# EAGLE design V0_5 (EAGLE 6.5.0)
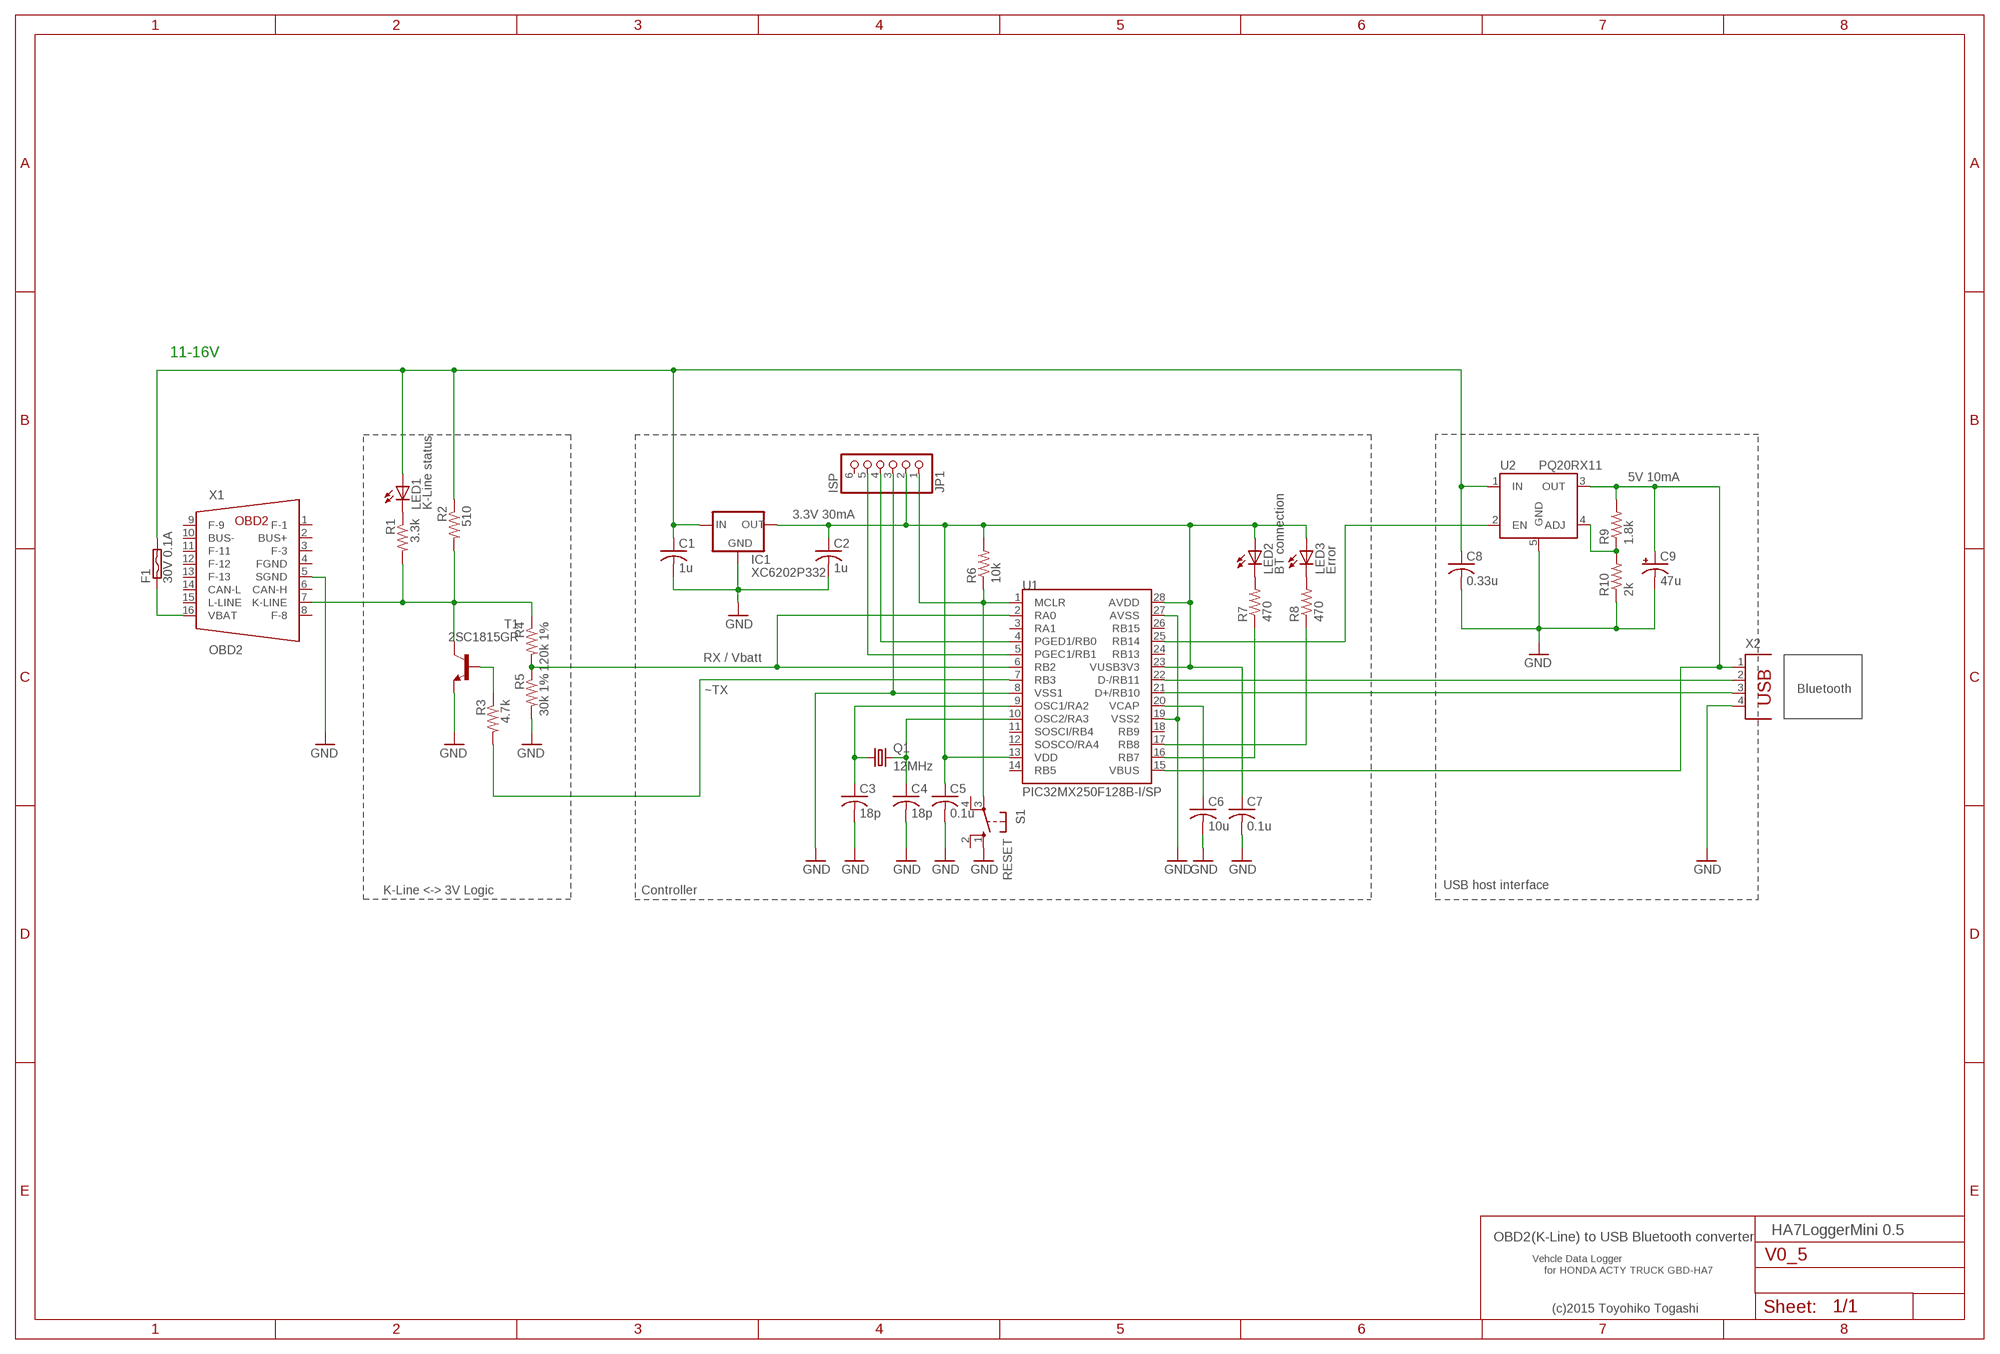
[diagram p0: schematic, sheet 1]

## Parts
C1  1u  C-US025-024X044  [C025-024X044]
C2  1u  C-US025-024X044  [C025-024X044]
C3  18p  C-US025-024X044  [C025-024X044]
C4  18p  C-US025-024X044  [C025-024X044]
C5  0.1u  C-US025-024X044  [C025-024X044]
C6  10u  C-US025-024X044  [C025-024X044]
C7  0.1u  C-US025-024X044  [C025-024X044]
C8  0.33u  C-US025-024X044  [C025-024X044]
C9  47u  CPOL-USE2.5-7  [E2,5-7]
F1  30V 0.1A  SMDH120  [SMD050F]
IC1  XC6202P332  78LXX  [78LXX]
JP1  ISP  PINHD-1X6  [1X06]
LED1  K-Line status  LED3MM  [LED3MM]
LED2  BT connection  LED3MM  [LED3MM]
LED3  Error  LED3MM  [LED3MM]
Q1  12MHz  CRYSTALHC49S  [HC49/S]
R1  3.3k  R-US_0204/5  [0204/5]
R2  510  R-US_0204/7  [0204/7]
R3  4.7k  R-US_0204/5  [0204/5]
R4  120k 1%  R-US_0204/7  [0204/7]
R5  30k 1%  R-US_0204/7  [0204/7]
R6  10k  R-US_0204/5  [0204/5]
R7  470  R-US_0204/5  [0204/5]
R8  470  R-US_0204/5  [0204/5]
R9  1.8k  R-US_0204/5  [0204/5]
R10  2k  R-US_0204/5  [0204/5]
S1  RESET  10-XX  [B3F-10XX]
T1  2SC1815GR  -NPN-TO92-ECB  [TO92-ECB]
U1  PIC32MX250F128B-I/SP  [DIL28-3]
U2  PQ20RX11  [L200S]
X1  OBD2  [2X08]
X2  PN87520  [PN87520]

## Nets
+5V: C9.+ R9.2 U1.15(VBUS) U2.3(OUT) X2.1
GND: C1.2 C2.2 C3.2 C4.2 C5.2 C6.2 C7.2 C8.2 C9.- IC1.GND JP1.3 R5.2 R10.1 S1.1(S) T1.E U1.8(VSS1) U1.19(VSS2) U1.27(AVSS) U2.5(GND) X1.5(SGND) X2.4
N$1: C3.1 Q1.1 U1.9(OSC1/RA2)
N$2: C4.1 Q1.2 U1.10(OSC2/RA3)
N$3: R7.1 U1.16(RB7)
N$4: JP1.4 U1.4(PGED1/RB0)
N$5: R3.2 U1.7(RB3)
N$6: R3.1 T1.B
N$7: JP1.5 U1.5(PGEC1/RB1)
N$8: C6.1 U1.20(VCAP)
N$9: U1.22(D-/RB11) X2.2
N$10: U1.21(D+/RB10) X2.3
N$11: LED2.K(C) R7.2
N$12: JP1.1 R6.1 S1.3(P) U1.1(MCLR)
N$15: LED3.K(C) R8.2
N$17: R8.1 U1.17(RB8)
N$18: F1.1 X1.16(VBAT)
N$20: R1.2 R2.2 R4.1 T1.C X1.7(K-LINE)
N$21: R4.2 R5.1 U1.2(RA0) U1.6(RB2)
N$22: LED1.K(C) R1.1
N$23: R9.1 R10.2 U2.4(ADJ)
N$24: U1.25(RB14) U2.2(EN)
N$26: C1.1 C8.1 F1.2 IC1.IN LED1.A R2.1 U2.1(IN)
N$32: C2.1 C5.1 C7.1 IC1.OUT JP1.2 LED2.A LED3.A R6.2 U1.13(VDD) U1.23(VUSB3V3) U1.28(AVDD)
Unconnected: JP1.6 S1.2(S1) S1.4(P1) U1.3(RA1) U1.11(SOSCI/RB4) U1.12(SOSCO/RA4) U1.14(RB5) U1.18(RB9) U1.24(RB13) U1.26(RB15) X1.1(F-1) X1.2(BUS+) X1.3(F-3) X1.6(CAN-H) X1.8(F-8) X1.9(F-9) X1.10(BUS-) X1.11(F-11) X1.12(F-12) X1.13(F-13) X1.14(CAN-L) X1.15(L-LINE)

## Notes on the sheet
- 11-16V
- 5V 10mA
- 3.3V 30mA
- RX / Vbatt
- ~TX | Bluetooth
- USB host interface
- K-Line <-> 3V Logic | Controller
- HA7LoggerMini 0.5
- OBD2(K-Line) to USB Bluetooth converter
- Vehcle Data Logger
- for HONDA ACTY TRUCK GBD-HA7
- (c)2015 Toyohiko Togashi

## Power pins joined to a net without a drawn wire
FGND: X1.4(FGND)

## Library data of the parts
C1-C8 = rcl:C-US: CAPACITOR, American symbol
C9 = rcl:CPOL-US: POLARIZED CAPACITOR, American symbol
F1 = switch-raychem:SMDH120: PolySwitch (TM) Resettable Device
IC1 = v-reg:78LXX: VOLTAGE REGULATOR
JP1 = pinhead:PINHD-1X6: PIN HEADER
LED1-LED3 = led:LED: LED
Q1 = crystal:CRYSTAL: CRYSTAL; OC_FARNELL: 1667008; OC_NEWARK: unknown
R1-R10 = rcl:R-US_: RESISTOR, American symbol
S1 = switch-omron:10-XX: OMRON SWITCH; MPN: B3F-1000; OC_FARNELL: 176432; OC_NEWARK: 36M3542
T1 = transistor:*-NPN-: NPN Transistror BF959 corrected 2008.03.06
U1 = TOG.rpt:PIC32MX250F128B
U2 = TOG:PQ20RX
X1 = TOG:OBD2: OBD2 Connecter
X2 = con-berg:PN87520: BERG USB connector; OC_FARNELL: unknown; OC_NEWARK: unknown

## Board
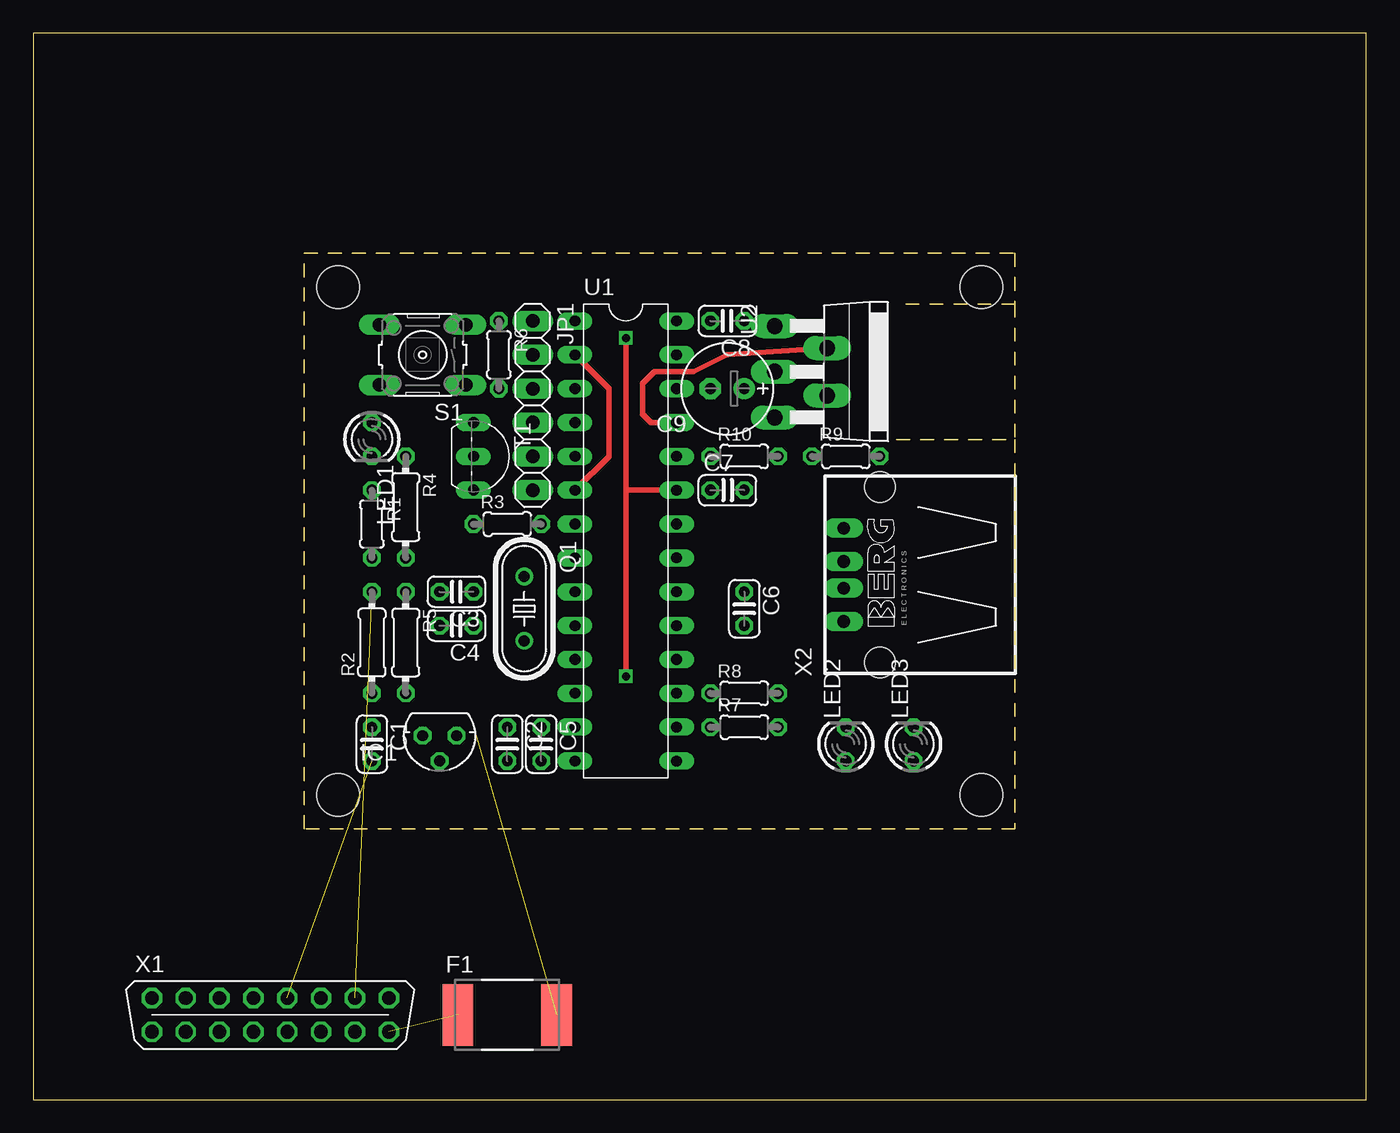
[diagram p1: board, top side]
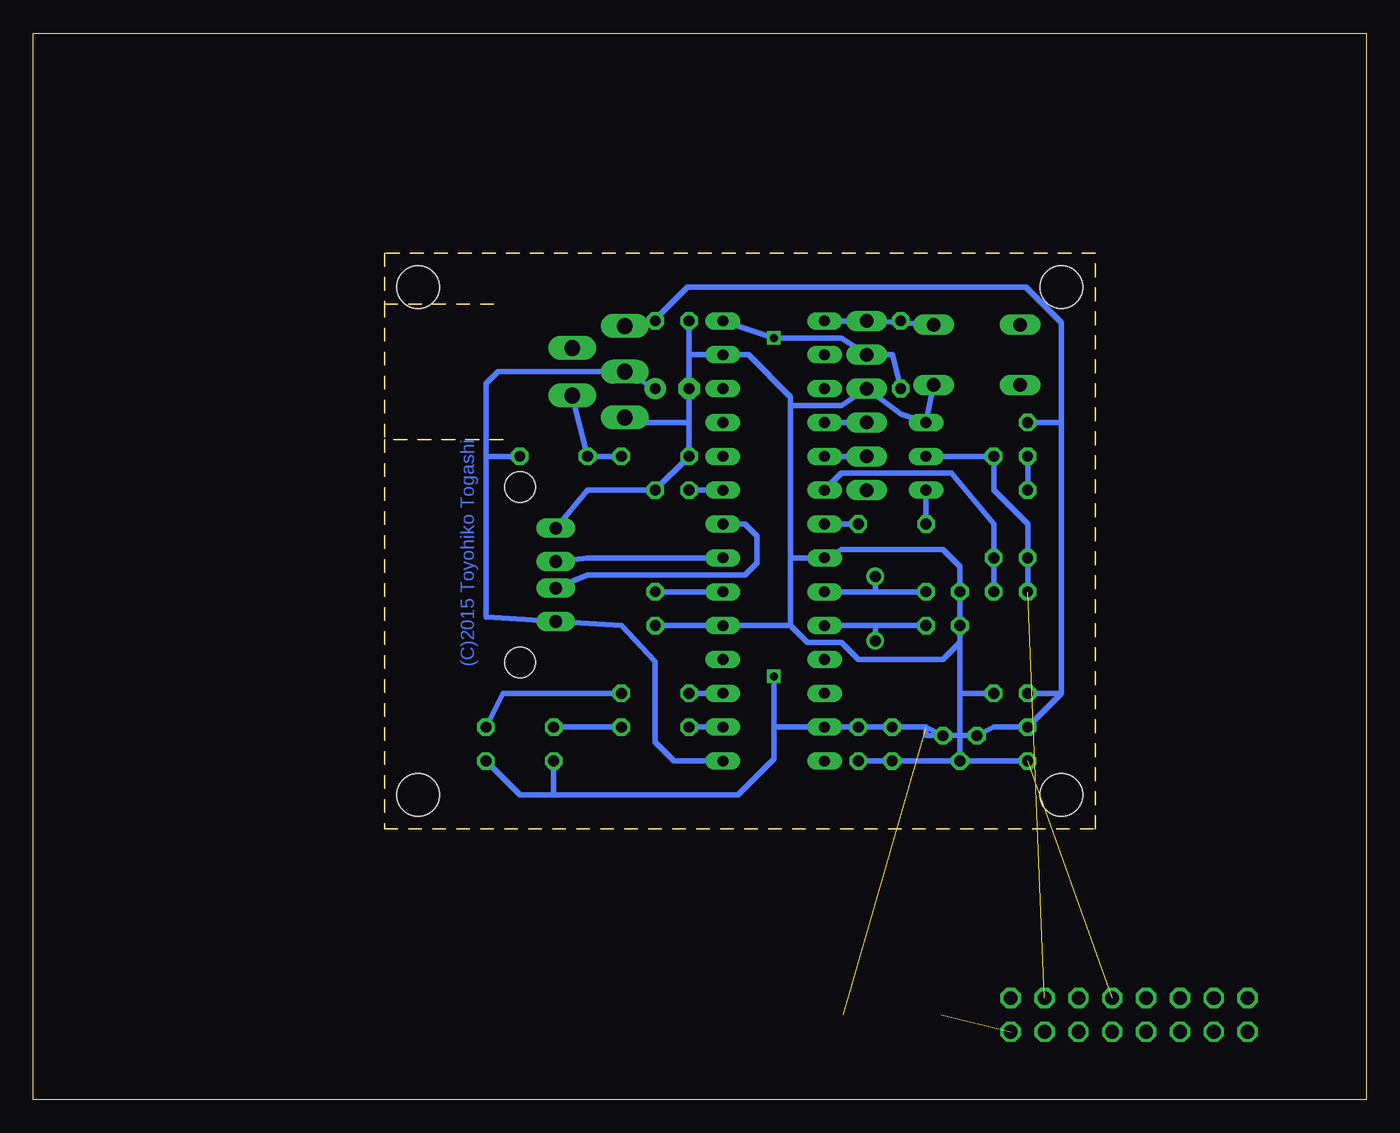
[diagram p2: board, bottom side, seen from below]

Size 100 x 80 mm. Coordinates in mm from the lower left corner, seen from the top.
Outline: 64.77,49.53 73.66,49.53
Outline: 73.66,59.69 64.77,59.69
Outline: 73.66,59.69 73.66,63.5 20.32,63.5 20.32,20.32 73.66,20.32 73.66,49.53
Outline: 73.66,59.69 73.66,49.53
Outline: 0,0 100,0 100,80 0,80 0,0
Copper layers (1*16): Top 0.035mm / dielectric 1.5mm / Bottom 0.035mm
Design rules "default": minimum track width 10mil, minimum drill 24mil, track to track 8mil, track to pad 8mil, pad to pad 8mil, via to via 8mil, smd to smd 8mil, copper to edge 40mil, drill to drill 8mil, minimum pad ring 10mil, minimum via ring 8mil, stop-mask expansion 4mil, vias tented up to drill 0mil, thermal gap 10mil
Holes 3.2 mm at 71.12,22.86 71.12,60.96 22.86,22.86 22.86,60.96

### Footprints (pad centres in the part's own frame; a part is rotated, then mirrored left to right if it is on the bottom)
C025-024X044 = drill 0.813 octagon: 1 -1.27,0; 2 1.27,0
E2,5-7 = drill 0.813 pad 1.6: + -1.27,0 | drill 0.813 pad 1.6 octagon: - 1.27,0
SMD050F = smd 2.3 x 4.6: 1 -3.7,0; 2 3.7,0
78LXX = drill 0.813 octagon: GND 0,1.905; IN 1.27,0; OUT -1.27,0
1X06 = drill 1.016 long: 1 -6.35,0; 2 -3.81,0; 3 -1.27,0; 4 1.27,0; 5 3.81,0; 6 6.35,0
LED3MM = drill 0.813 octagon: A -1.27,0; K 1.27,0
HC49/S = drill 0.813: 1 -2.413,0; 2 2.413,0
0204/5 = drill 0.813 octagon: 1 -2.54,0; 2 2.54,0
0204/7 = drill 0.813 octagon: 1 -3.81,0; 2 3.81,0
B3F-10XX = drill 1.016 long: 1 -3.251,2.261; 2 3.251,2.261; 3 -3.251,-2.261; 4 3.251,-2.261
TO92-ECB = drill 0.813 long: B 2.54,0; C 0,0; E -2.54,0
DIL28-3 = drill 0.8 long: 1 -16.51,-3.81; 2 -13.97,-3.81; 3 -11.43,-3.81; 4 -8.89,-3.81; 5 -6.35,-3.81; 6 -3.81,-3.81; 7 -1.27,-3.81; 8 1.27,-3.81; 9 3.81,-3.81; 10 6.35,-3.81; 11 8.89,-3.81; 12 11.43,-3.81; 13 13.97,-3.81; 14 16.51,-3.81; 15 16.51,3.81; 16 13.97,3.81; 17 11.43,3.81; 18 8.89,3.81; 19 6.35,3.81; 20 3.81,3.81; 21 1.27,3.81; 22 -1.27,3.81; 23 -3.81,3.81; 24 -6.35,3.81; 25 -8.89,3.81; 26 -11.43,3.81; 27 -13.97,3.81; 28 -16.51,3.81
L200S = drill 1.194 long: 1 -3.429,-8.509; 2 -1.778,-4.572; 3 0,-8.509; 4 1.778,-4.572; 5 3.429,-8.509
2X08 = drill 1.016 octagon: 1 -8.89,1.27; 2 -6.35,1.27; 3 -1.27,1.27; 4 -3.81,1.27; 5 1.27,1.27; 6 3.81,1.27; 7 6.35,1.27; 8 8.89,1.27; 9 -8.89,-1.27; 10 -6.35,-1.27; 11 -3.81,-1.27; 12 -1.27,-1.27; 13 1.27,-1.27; 14 3.81,-1.27; 15 6.35,-1.27; 16 8.89,-1.27
PN87520 = drill 0.95 long: 1 -3.5,2.71; 2 -1,2.71; 3 1,2.71; 4 3.5,2.71 | hole 2.3: -6.57,0; 6.57,0

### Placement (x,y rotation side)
C1  25.4,26.67 270 top
C2  35.56,26.67 270 top
C3  31.75,38.1 180 top
C4  31.75,35.56 180 top
C5  38.1,26.67 270 top
C6  53.34,36.83 270 top
C7  52.07,45.72 0 top
C8  52.07,58.42 180 top
C9  52.07,53.34 180 top
F1  35.56,6.35 0 top
IC1  30.48,27.3 180 top
JP1  37.47,52.07 270 top
LED1  25.4,49.53 270 top
LED2  60.96,26.67 90 top
LED3  66.04,26.67 90 top
Q1  36.83,36.83 270 top
R1  25.4,43.18 270 top
R2  25.4,34.29 90 top
R3  35.56,43.18 0 top
R4  27.94,44.45 270 top
R5  27.94,34.29 270 top
R6  34.92,55.88 270 top
R7  53.34,27.94 0 top
R8  53.34,30.48 0 top
R9  60.96,48.26 0 top
R10  53.34,48.26 0 top
S1  29.21,55.88 180 top
T1  33.02,48.26 270 top
U1  44.45,41.91 270 top
U2  64.14,54.61 270 top
X1  17.78,6.35 0 top
X2  63.5,39.37 90 top

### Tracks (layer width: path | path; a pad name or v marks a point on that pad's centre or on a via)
+5V
  Bottom 0.406: C9.+ U2.3 65.14,54.61 66.04,53.71 66.04,48.26 | 66.04,48.26 66.04,36.2 X2.1 55.88,35.56 53.34,32.87 53.34,26.82 51.92,25.4 U1.15 | R9.2 66.04,48.26
GND  (1 unrouted)
  Bottom 0.406: 43.18,35.56 43.18,40.64 | 43.18,35.56 U1.19 C6.2 | IC1.GND C2.2 C5.2 | U2.5 54.61,50.8 50.8,50.8 | X2.4 58.42,45.72 C7.2 R10.1 50.8,50.8 | IC1.GND C1.2 | 43.18,40.64 U1.8 39.37,41.27 31.75,41.27 30.48,40.01 C3.2 C4.2 30.48,34.29 | 43.18,35.56 41.91,34.29 39.37,34.29 38.1,33.02 31.75,33.02 30.48,34.29 | S1.1 T1.E 34.92,51.44 JP1.3 39.37,52.07 43.18,52.07 | 50.8,55.88 U1.27 46.35,55.88 43.18,52.7 43.18,52.07 | 50.8,58.67 C8.2 50.8,55.88 | 43.18,40.64 43.18,52.07 | 50.8,55.88 C9.- 50.8,50.8 | IC1.GND 30.48,30.48 | R5.2 30.48,30.48 | 30.48,34.29 30.48,30.48
N$1
  Bottom 0.406: C3.1 36.83,38.1 | 36.83,38.1 U1.9 | Q1.1 36.83,38.1
N$2
  Bottom 0.406: U1.10 36.83,35.56 | 36.83,35.56 C4.1 | Q1.2 36.83,35.56
N$3
  Bottom 0.406: R7.1 U1.16
N$4
  Bottom 0.406: U1.4 JP1.4
N$5
  Bottom 0.406: U1.7 R3.2
N$6
  Bottom 0.406: R3.1 T1.B
N$7
  Bottom 0.406: U1.5 JP1.5
N$8
  Bottom 0.406: U1.20 C6.1
N$9
  Bottom 0.406: X2.2 58.42,39.37 46.62,39.37 45.72,40.27 45.72,42.28 46.62,43.18 U1.22
N$10
  Bottom 0.406: X2.3 58.42,40.64 U1.21
N$11
  Bottom 0.406: R7.2 LED2.K
N$12
  Bottom 0.406: U1.1 JP1.1 35.57,58.31 | S1.3 35.57,58.31 | R6.1 35.57,58.31
N$15
  Bottom 0.406: R8.2 64.77,30.48 LED3.K
N$17
  Bottom 0.406: R8.1 U1.17
N$18  (1 unrouted)
N$20  (1 unrouted)
  Bottom 0.406: T1.C R4.1 27.94,45.72 25.4,43.18 R1.2 R2.2
N$21
  Top 0.406: U1.2 43.18,53.34 43.18,48.26 U1.6
  Bottom 0.406: R5.1 R4.2 27.94,43.18 31.11,46.99 39.37,46.99 U1.6
N$22
  Bottom 0.406: LED1.K R1.1
N$23
  Bottom 0.406: U2.4 R9.1 R10.2
N$24
  Top 0.406: U1.25 46.35,50.8 45.72,51.44 45.72,53.71 46.62,54.61 49.53,54.61 52.07,55.88 U2.2
N$26  (1 unrouted)
  Bottom 0.406: U2.1 C8.1 53.34,58.53 50.91,60.96 25.53,60.96 22.86,58.29 22.86,50.8 | 22.86,30.48 22.86,50.8 | LED1.A 22.86,50.8 | 22.86,30.48 C1.1 27.94,27.94 IC1.IN 33.02,27.3 33.02,27.94 | R2.1 22.86,30.48
N$32  (via drill 0.6)
  Top 0.406: v44.45,31.75 44.45,45.72 | U1.23 44.45,45.72 | 44.45,45.72 v44.45,57.15
  Bottom 0.406: IC1.OUT 33.02,27.94 C2.1 C5.1 U1.13 44.45,27.94 | U1.23 C7.1 | 44.45,27.94 v44.45,31.75 | U1.28 v44.45,57.15 39.37,57.15 JP1.2 35.56,55.88 R6.2 | 44.45,27.94 44.45,25.55 47.14,22.86 60.96,22.86 | 60.96,22.86 63.5,22.86 LED3.A | LED2.A 60.96,22.86

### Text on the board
Bottom: (C)2015 Toyohiko Togashi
